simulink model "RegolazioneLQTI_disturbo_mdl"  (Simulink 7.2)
settings: Solver=ode45  StartTime=0.0  StopTime=10.0  RelTol=1e-3
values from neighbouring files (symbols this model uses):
  A = [0 1; -2 1]    [RegolazioneOttimaTempoInfinita_Integrale.m]    (also in RegolazioneOttimaTempoInfinita_TempoDiscreto.m; RegolazioneOttimaTempoInfinita_uscita.m; RegolazioneOttimaTempoInfinita_uscita_osservatore.m; RegolazioneOttimaTempoInfinita.m)
  B = [0; 1]    [RegolazioneOttimaTempoInfinita_Integrale.m]    (also in RegolazioneOttimaTempoInfinita_TempoDiscreto.m; RegolazioneOttimaTempoInfinita_uscita.m; RegolazioneOttimaTempoInfinita_uscita_osservatore.m; RegolazioneOttimaTempoInfinita.m)
  S1A = 0    [RegolazioneOttimaTempoInfinita_Integrale.m]    (also in RegolazioneOttimaTempoInfinita_uscita.m; RegolazioneOttimaTempoInfinita.m)
  S1T = 5    [RegolazioneOttimaTempoInfinita_Integrale.m]    (also in RegolazioneOttimaTempoInfinita_uscita.m; RegolazioneOttimaTempoInfinita.m)
  S2A = 1    [RegolazioneOttimaTempoInfinita_Integrale.m]    (also in RegolazioneOttimaTempoInfinita_uscita.m; RegolazioneOttimaTempoInfinita.m)
  S2T = 5    [RegolazioneOttimaTempoInfinita_Integrale.m]    (also in RegolazioneOttimaTempoInfinita_uscita.m; RegolazioneOttimaTempoInfinita.m)
  X0 = [2;-3]    [RegolazioneOttimaTempoInfinita_Integrale.m]    (also in RegolazioneOttimaTempoInfinita_TempoDiscreto.m; RegolazioneOttimaTempoInfinita_uscita.m; RegolazioneOttimaTempoInfinita_uscita_osservatore.m; RegolazioneOttimaTempoInfinita.m)
undefined symbols (not defined in the file or in its folder): K

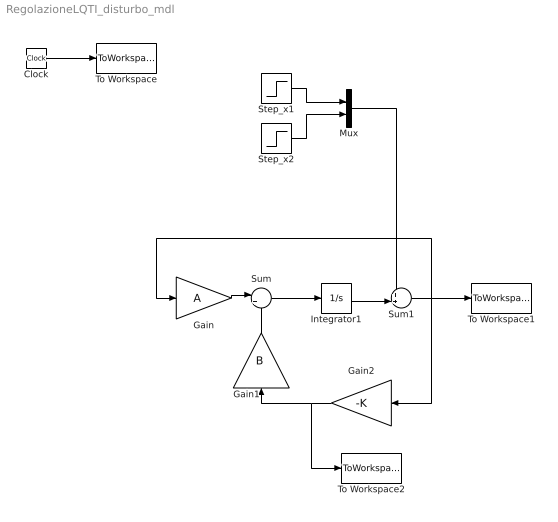
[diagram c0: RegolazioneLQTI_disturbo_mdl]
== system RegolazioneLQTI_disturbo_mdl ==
  Clock : Clock
  Gain : Gain  Gain=A  Multiplication=Matrix(K*u)  ParameterDataType=sfix(16)  ParameterScaling=2^0  OutDataType=sfix(16)  OutScaling=2^0
  Gain1 : Gain  Orientation=up  Gain=B  Multiplication=Matrix(K*u)  ParameterDataType=sfix(16)  ParameterScaling=2^0  OutDataType=sfix(16)  OutScaling=2^0
  Gain2 : Gain  Orientation=left  Gain=-K  Multiplication=Matrix(K*u)  ParameterDataType=sfix(16)  ParameterScaling=2^0  OutDataType=sfix(16)  OutScaling=2^0
  Integrator1 : Integrator  InitialCondition=X0
  Mux : Mux  Inputs=2
  Step_x1 : Step  Time=S1T  After=S1A  SampleTime=0
  Step_x2 : Step  Time=S2T  After=S2A  SampleTime=0
  Sum : Sum  Inputs=|++  OutDataType=sfix(16)  OutScaling=2^0
  Sum1 : Sum  Inputs=++|  OutDataType=sfix(16)  OutScaling=2^0
  To Workspace : ToWorkspace  VariableName=time  SampleTime=-1  SaveFormat=Array
  To Workspace1 : ToWorkspace  VariableName=X  SampleTime=-1  SaveFormat=Array
  To Workspace2 : ToWorkspace  VariableName=u  SampleTime=-1  SaveFormat=Array
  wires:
  Gain/1 -> Sum/1
  Sum1/1 -> Gain/1, Gain2/1, To Workspace1/1
  Gain1/1 -> Sum/2
  Gain2/1 -> Gain1/1, To Workspace2/1
  Sum/1 -> Integrator1/1
  Clock/1 -> To Workspace/1
  Integrator1/1 -> Sum1/2
  Step_x1/1 -> Mux/1
  Step_x2/1 -> Mux/2
  Mux/1 -> Sum1/1
